FUNCTION_BLOCK FB_SignalHandlingDelay EXTENDS FB_SignalHandling
VAR_INPUT
	tDelay			: TIME;
END_VAR
VAR
	bSet			: BOOL;
	fbTimerDelay	: TON;
END_VAR

// =========================================================
;
// =========================================================

METHOD PUBLIC M_SetOutput
VAR_INPUT
END_VAR
// =========================================================
	// Out

IF bEnable AND bInput THEN
	bSet := TRUE;
END_IF

IF bSet THEN
	fbTimerDelay(	IN := TRUE,
					PT := tDelay);
ELSE
	fbTimerDelay(	IN := FALSE);
END_IF

IF fbTimerDelay.Q THEN
	bSet := FALSE;
	
	fbTimerDelay(IN := FALSE);
	
	bOut := TRUE;
ELSE
	bOut := FALSE;
END_IF
			
// =========================================================
END_METHOD

END_FUNCTION_BLOCK
